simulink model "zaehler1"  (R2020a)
settings: Solver=FixedStepDiscrete  StartTime=0.0  StopTime=Inf  FixedStep=1e-6  RelTol=1e-3  EnableMultiTasking=on

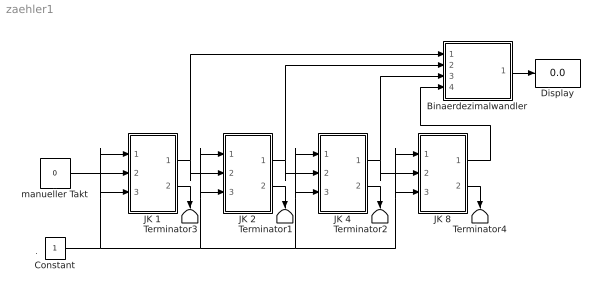
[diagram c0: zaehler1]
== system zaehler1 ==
  note: .
  Binaerdezimalwandler : Subsystem
  Constant : Constant
  Display : Display
  JK 1 : Subsystem  mask(JKFlipFlop){initial_condition=0}
      mask prompts: initial_condition "Initial condition (state of Q):"
      mask help: J-K Flip-Flop Block (Negative Edge Triggered)
  JK 2 : Subsystem  mask(JKFlipFlop){initial_condition=0}
      mask prompts: initial_condition "Initial condition (state of Q):"
      mask help: J-K Flip-Flop Block (Negative Edge Triggered)
  JK 4 : Subsystem  mask(JKFlipFlop){initial_condition=0}
      mask prompts: initial_condition "Initial condition (state of Q):"
      mask help: J-K Flip-Flop Block (Negative Edge Triggered)
  JK 8 : Subsystem  mask(JKFlipFlop){initial_condition=0}
      mask prompts: initial_condition "Initial condition (state of Q):"
      mask help: J-K Flip-Flop Block (Negative Edge Triggered)
  Terminator{1..4} (4 alike) : Terminator
  manueller Takt : Constant  Value=0
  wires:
  JK 4/1(Q) -> Binaerdezimalwandler/3(In4), JK 8/2(CLK)
  JK 2/1(Q) -> Binaerdezimalwandler/2(In2), JK 4/2(CLK)
  JK 1/1(Q) -> Binaerdezimalwandler/1(In1), JK 2/2(CLK)
  manueller Takt/1 -> JK 1/2(CLK)
  Constant/1 -> JK 2/3(K), JK 2/1(J), JK 4/3(K), JK 4/1(J), JK 8/1(J), JK 8/3(K), JK 1/1(J), JK 1/3(K)
  JK 8/1(Q) -> Binaerdezimalwandler/4(In8)
  Binaerdezimalwandler/1(Out) -> Display/1
  JK 1/2(!Q) -> Terminator3/1
  JK 2/2(!Q) -> Terminator1/1
  JK 4/2(!Q) -> Terminator2/1
  JK 8/2(!Q) -> Terminator4/1

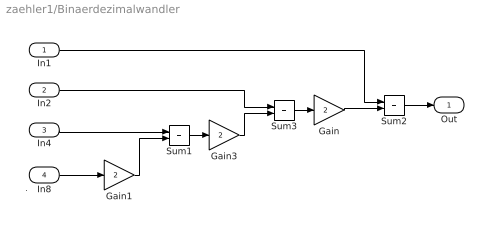
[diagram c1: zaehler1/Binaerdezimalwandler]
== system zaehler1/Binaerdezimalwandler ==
  note: .
  In1 : Inport
  In2 : Inport  Port=2
  In4 : Inport  Port=3
  In8 : Inport  Port=4
  Gain : Gain  Gain=2  SaturateOnIntegerOverflow=on
  Gain1 : Gain  Gain=2  SaturateOnIntegerOverflow=on
  Gain3 : Gain  Gain=2  SaturateOnIntegerOverflow=on
  Sum1 : Sum  SaturateOnIntegerOverflow=on
  Sum2 : Sum  SaturateOnIntegerOverflow=on
  Sum3 : Sum  SaturateOnIntegerOverflow=on
  Out : Outport
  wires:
  Gain/1 -> Sum2/2
  In1/1 -> Sum2/1
  Sum2/1 -> Out/1
  Sum3/1 -> Gain/1
  In2/1 -> Sum3/1
  Gain3/1 -> Sum3/2
  Sum1/1 -> Gain3/1
  In4/1 -> Sum1/1
  Gain1/1 -> Sum1/2
  In8/1 -> Gain1/1

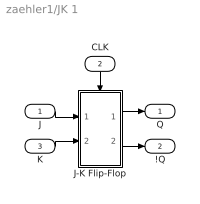
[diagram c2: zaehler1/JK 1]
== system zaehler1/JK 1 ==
  J : Inport
  CLK : Inport  Port=2
  K : Inport  Port=3
  J-K Flip-Flop : Subsystem  TreatAsAtomicUnit=on
  Q : Outport
  !Q : Outport  Port=2
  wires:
  CLK/1 -> J-K Flip-Flop/Trigger
  J-K Flip-Flop/1(Q) -> Q/1
  J/1 -> J-K Flip-Flop/1(J)
  K/1 -> J-K Flip-Flop/2(K)
  J-K Flip-Flop/2(!Q) -> !Q/1

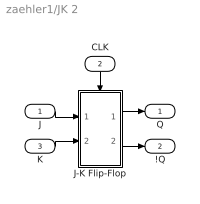
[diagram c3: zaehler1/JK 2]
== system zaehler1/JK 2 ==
  J : Inport
  CLK : Inport  Port=2
  K : Inport  Port=3
  J-K Flip-Flop : Subsystem  TreatAsAtomicUnit=on
  Q : Outport
  !Q : Outport  Port=2
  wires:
  CLK/1 -> J-K Flip-Flop/Trigger
  J-K Flip-Flop/1(Q) -> Q/1
  J/1 -> J-K Flip-Flop/1(J)
  K/1 -> J-K Flip-Flop/2(K)
  J-K Flip-Flop/2(!Q) -> !Q/1

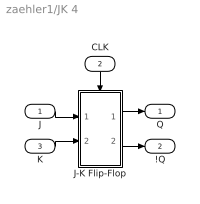
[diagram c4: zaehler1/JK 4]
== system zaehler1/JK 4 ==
  J : Inport
  CLK : Inport  Port=2
  K : Inport  Port=3
  J-K Flip-Flop : Subsystem  TreatAsAtomicUnit=on
  Q : Outport
  !Q : Outport  Port=2
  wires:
  CLK/1 -> J-K Flip-Flop/Trigger
  J-K Flip-Flop/1(Q) -> Q/1
  J/1 -> J-K Flip-Flop/1(J)
  K/1 -> J-K Flip-Flop/2(K)
  J-K Flip-Flop/2(!Q) -> !Q/1

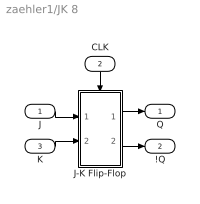
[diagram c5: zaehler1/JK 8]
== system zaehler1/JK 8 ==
  J : Inport
  CLK : Inport  Port=2
  K : Inport  Port=3
  J-K Flip-Flop : Subsystem  TreatAsAtomicUnit=on
  Q : Outport
  !Q : Outport  Port=2
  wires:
  CLK/1 -> J-K Flip-Flop/Trigger
  J-K Flip-Flop/1(Q) -> Q/1
  J/1 -> J-K Flip-Flop/1(J)
  K/1 -> J-K Flip-Flop/2(K)
  J-K Flip-Flop/2(!Q) -> !Q/1

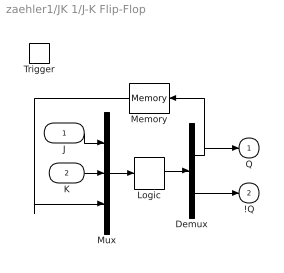
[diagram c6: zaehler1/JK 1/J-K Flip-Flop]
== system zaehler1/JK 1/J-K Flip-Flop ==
  J : Inport
  K : Inport  Port=2
  Trigger : TriggerPort  TriggerType=falling  VariantControl=Variant
  Demux : Demux  Outputs=2
  Logic : CombinatorialLogic  TruthTable=[0 1; 1 0; 0 1; 0 1; 1 0; 1 0; 1 0; 0 1]
  Memory : Memory  InitialCondition=initial_condition  InheritSampleTime=on
  Mux : Mux  Inputs=3
  Q : Outport  InitialOutput=initial_condition
  !Q : Outport  Port=2  InitialOutput=~initial_condition
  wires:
  Mux/1 -> Logic/1
  Logic/1 -> Demux/1
  Demux/2 -> !Q/1
  Demux/1 -> Memory/1, Q/1
  J/1 -> Mux/1
  K/1 -> Mux/2
  Memory/1 -> Mux/3

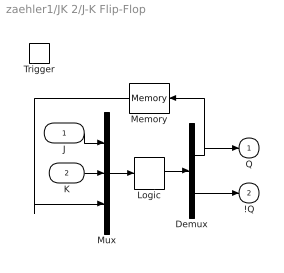
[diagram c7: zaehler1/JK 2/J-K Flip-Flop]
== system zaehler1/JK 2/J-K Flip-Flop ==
  J : Inport
  K : Inport  Port=2
  Trigger : TriggerPort  TriggerType=falling  VariantControl=Variant
  Demux : Demux  Outputs=2
  Logic : CombinatorialLogic  TruthTable=[0 1; 1 0; 0 1; 0 1; 1 0; 1 0; 1 0; 0 1]
  Memory : Memory  InitialCondition=initial_condition  InheritSampleTime=on
  Mux : Mux  Inputs=3
  Q : Outport  InitialOutput=initial_condition
  !Q : Outport  Port=2  InitialOutput=~initial_condition
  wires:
  Mux/1 -> Logic/1
  Logic/1 -> Demux/1
  Demux/2 -> !Q/1
  Demux/1 -> Memory/1, Q/1
  J/1 -> Mux/1
  K/1 -> Mux/2
  Memory/1 -> Mux/3

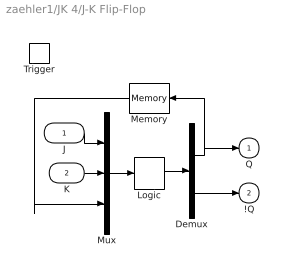
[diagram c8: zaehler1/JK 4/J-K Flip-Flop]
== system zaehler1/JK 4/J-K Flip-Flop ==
  J : Inport
  K : Inport  Port=2
  Trigger : TriggerPort  TriggerType=falling  VariantControl=Variant
  Demux : Demux  Outputs=2
  Logic : CombinatorialLogic  TruthTable=[0 1; 1 0; 0 1; 0 1; 1 0; 1 0; 1 0; 0 1]
  Memory : Memory  InitialCondition=initial_condition  InheritSampleTime=on
  Mux : Mux  Inputs=3
  Q : Outport  InitialOutput=initial_condition
  !Q : Outport  Port=2  InitialOutput=~initial_condition
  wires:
  Mux/1 -> Logic/1
  Logic/1 -> Demux/1
  Demux/2 -> !Q/1
  Demux/1 -> Memory/1, Q/1
  J/1 -> Mux/1
  K/1 -> Mux/2
  Memory/1 -> Mux/3

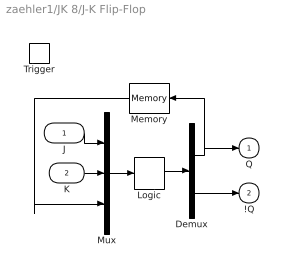
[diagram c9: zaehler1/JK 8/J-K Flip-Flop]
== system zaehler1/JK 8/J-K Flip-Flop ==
  J : Inport
  K : Inport  Port=2
  Trigger : TriggerPort  TriggerType=falling  VariantControl=Variant
  Demux : Demux  Outputs=2
  Logic : CombinatorialLogic  TruthTable=[0 1; 1 0; 0 1; 0 1; 1 0; 1 0; 1 0; 0 1]
  Memory : Memory  InitialCondition=initial_condition  InheritSampleTime=on
  Mux : Mux  Inputs=3
  Q : Outport  InitialOutput=initial_condition
  !Q : Outport  Port=2  InitialOutput=~initial_condition
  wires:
  Mux/1 -> Logic/1
  Logic/1 -> Demux/1
  Demux/2 -> !Q/1
  Demux/1 -> Memory/1, Q/1
  J/1 -> Mux/1
  K/1 -> Mux/2
  Memory/1 -> Mux/3
